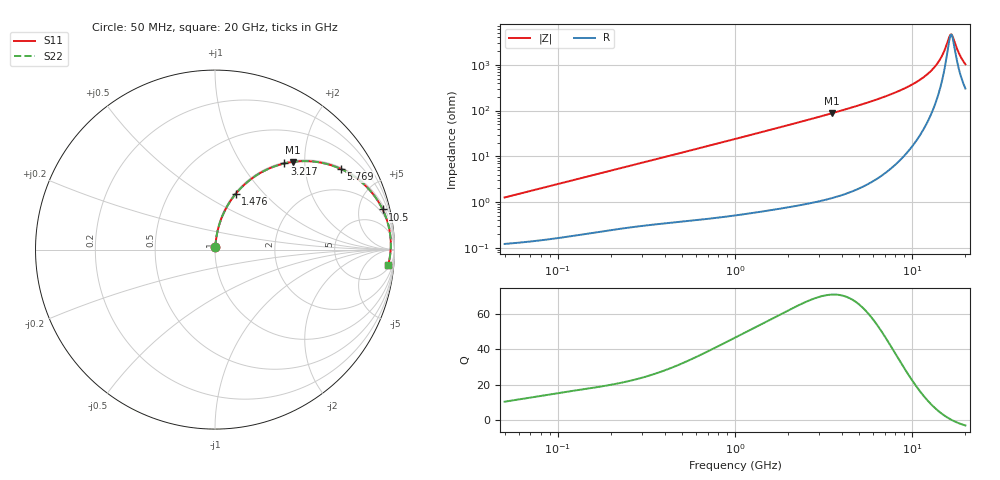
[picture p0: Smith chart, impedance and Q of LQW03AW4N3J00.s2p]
!Murata Part Number: LQW03AW4N3J00
!These Parameters are Measured in Series Mode Connection
!  o--[Z]--o
!Port1  Port2
!  o-------o
!Freq. Start=50[MHz] Stop=20[GHz], 401[Steps]
# Hz S RI R 50
!Freq.(Hz) S11(Real) S11(Imag) S21(Real) S21(Imag) S12(Real) S12(Imag) S22(Real) S22(Imag)
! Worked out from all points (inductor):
!   401 points, 50 MHz to 20 GHz, reference 50 ohm
!   read as one part in series: L = 4 nH near 51.52 MHz
!   highest Q = 71.2 at 3.519 GHz (marker M1), where L = 3.94 nH
!   self-resonance near 16.46 GHz
!   S11 on the Smith chart (normalised r, x): 50 MHz: 1.00, +0.03; 1.476 GHz: 1.01, +0.71; 3.217 GHz: 1.02, +1.58; 5.769 GHz: 1.05, +3.10; 10.5 GHz: 1.43, +8.23; 20 GHz: 7, -20
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5e7  0.00138 0.0126  0.9986 -0.0126  0.9986 -0.0126  0.00138 0.0126
1.364002e8  0.00309 0.0336  0.9969 -0.0336  0.9969 -0.0336  0.00309 0.0336
3.721004e8  0.0113 0.0886  0.9887 -0.0886  0.9887 -0.0886  0.0113 0.0886
1e9  0.0585 0.2242  0.9415 -0.2242  0.9415 -0.2242  0.0585 0.2242
1.476162e9  0.1156 0.3108  0.8844 -0.3108  0.8844 -0.3108  0.1156 0.3108
2.021818e9  0.1953 0.3885  0.8047 -0.3885  0.8047 -0.3885  0.1953 0.3885
2.728004e9  0.3083 0.4546  0.6917 -0.4546  0.6917 -0.4546  0.3083 0.4546
3.216634e9  0.3861 0.4798  0.6139 -0.4798  0.6139 -0.4798  0.3861 0.4798
3.519108e9  0.4324 0.4884  0.5676 -0.4884  0.5676 -0.4884  0.4324 0.4884
4.539627e9  0.5722 0.4875  0.4278 -0.4875  0.4278 -0.4875  0.5722 0.4875
5.769027e9  0.7027 0.4487  0.2973 -0.4487  0.2973 -0.4487  0.7027 0.4487
7.442007e9  0.8227 0.3705  0.1773 -0.3705  0.1773 -0.3705  0.8227 0.3705
1.050288e10  0.9341 0.2237  0.0659 -0.2237  0.0659 -0.2237  0.9341 0.2237
1.220001e10  0.9617 0.1521  0.0383 -0.1521  0.0383 -0.1521  0.9617 0.1521
1.375312e10  0.9746 0.0935  0.0254 -0.0935  0.0254 -0.0935  0.9746 0.0935
1.482269e10  0.9787 0.0568  0.0213 -0.0568  0.0213 -0.0568  0.9787 0.0568
1.597544e10  0.9796 0.0201  0.0204 -0.0201  0.0204 -0.0201  0.9796 0.0201
1.646126e10  0.9791 0.00554  0.0209 -0.00554  0.0209 -0.00554  0.9791 0.00554
1.696185e10  0.9781 -0.00899  0.0219 0.00899  0.0219 0.00899  0.9781 -0.00899
1.855685e10  0.9723 -0.0521  0.0277 0.0521  0.0277 0.0521  0.9723 -0.0521
1.940974e10  0.9678 -0.0733  0.0322 0.0733  0.0322 0.0733  0.9678 -0.0733
2e10  0.9641 -0.0873  0.0359 0.0873  0.0359 0.0873  0.9641 -0.0873
